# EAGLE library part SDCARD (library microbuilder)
SD Card Reader 06132 = Inexpensive SMT 19646 = Push/Pull SMT
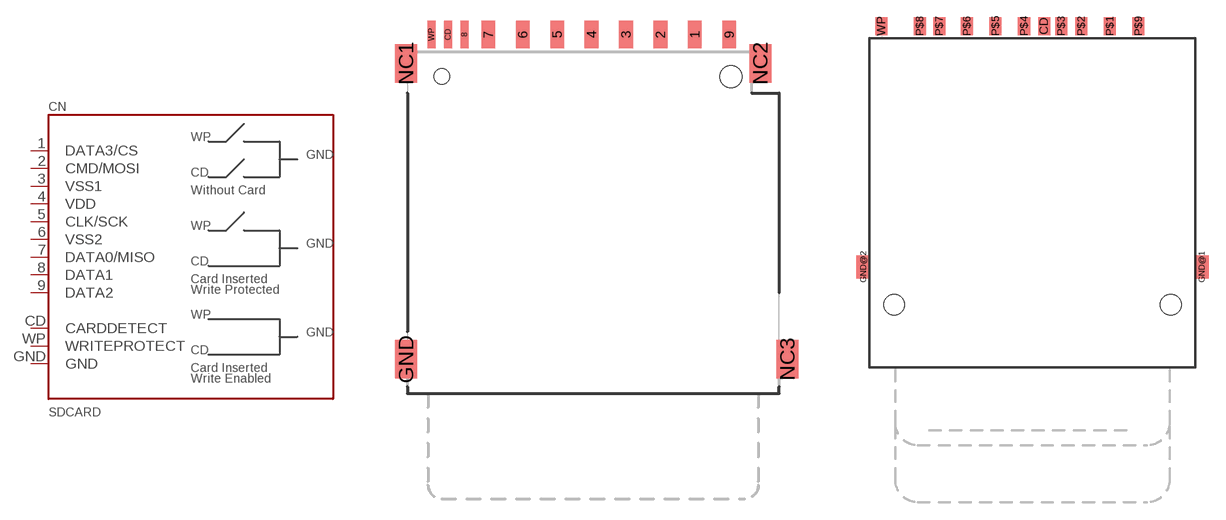
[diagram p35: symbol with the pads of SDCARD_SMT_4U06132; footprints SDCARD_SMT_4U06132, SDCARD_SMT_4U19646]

Designator prefix CN

## SDCARD  [SDCARD_SMT_4U06132]
1  DATA3/CS
2  CMD/MOSI
3  VSS1
4  VDD
5  CLK/SCK
6  VSS2
7  DATA0/MISO
8  DATA1
9  DATA2
CD  CARDDETECT
GND  GND
WP  WRITEPROTECT

## SDCARD19646  [SDCARD_SMT_4U19646]
CD  CARDDETECT
GND@2  GND
P$1  DATA3/CS
P$2  CMD/MOSI
P$3  VSS1
P$4  VDD
P$5  CLK/SCK
P$6  VSS2
P$7  DATA0/MISO
P$8  DATA1
P$9  DATA2
WP  WRITEPROTECT

## Footprint SDCARD_SMT_4U06132 (pad centres in mm)
SD Card Holder - 90° SMT 4UConnector: 06132
smd 1 x 2.008: 1 6.88,11.254; 2 4.38,11.254; 3 1.88,11.254; 4 -0.62,11.254; 5 -3.12,11.254; 6 -5.62,11.254; 7 -8.12,11.254; 9 9.38,11.254
smd 0.6 x 2.008: 8 -9.845,11.254; CD -11.045,11.254; WP -12.245,11.254
smd 1.6 x 2.8: GND -14.1,-12.35; NC1 -14.1,9.15; NC2 11.631,9.15; NC3 13.6,-12.35
hole 1.6 at 9.5,8.2
hole 1.1 at -11.5,8.2

## Footprint SDCARD_SMT_4U19646 (pad centres in mm)
Push/Pull SD Connector - 4U 19646
smd 1.05 x 1.56: CD 1.02,15.47; P$1 6.77,15.47; P$2 4.27,15.47; P$3 2.52,15.47; P$4 -0.73,15.47; P$5 -3.23,15.47; P$6 -5.73,15.47; P$7 -8.15,15.47; P$8 -9.85,15.47; P$9 9.27,15.47; WP -13.2,15.47
smd 1.2 x 2: GND@1 14.8,-5.6; GND@2 -14.8,-5.6
hole 1.8 at -12.1,-8.9
hole 1.8 at 12.1,-8.9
